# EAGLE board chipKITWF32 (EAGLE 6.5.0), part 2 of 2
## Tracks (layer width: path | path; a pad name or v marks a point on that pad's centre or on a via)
AN2/C2IN-/CN4/RB2
  Bottom 0.203: R24.2 65.53,7.37 70.36,2.54 70.61,2.54 J8.1
AN3/C2IN+/CN5/RB3
  Bottom 0.203: R25.2 66.67,7.49 69.22,4.95 70.99,4.95 J8.2
AN4/C1IN-/CN6/RB4
  Bottom 0.203: R26.2 67.82,7.49 69.09,6.22 69.22,6.22 71.5,6.22 72.39,5.33 72.39,3.81 J8.3
AN5/C1IN+/VBUSON/CN7/RB5
  Top 0.127: JP11.2 71.37,15.24 74.55,12.06 75.82,12.06 76.45,11.43 76.45,10.16 76.71,9.91 76.71,8.13 J8.4
  Bottom 0.127: R27.2
  Bottom 0.203: R27.2 68.96,7.24 69.6,6.6 71.75,6.6 73.28,5.08 J8.4
AN8/C1OUT/RB8
  Bottom 0.203: R28.2 70.1,7.49 70.61,6.99 72.01,6.99 72.77,6.22 74.17,6.22 74.93,5.46 74.93,3.81 J8.5
AN9/C2OUT/RB9
  Bottom 0.203: R29.2 71.75,7.37 72.26,7.37 73.03,6.6 74.68,6.6 J8.6
AN10/CVREFOUT/PMA13/RB10
  Bottom 0.203: R30.2 53.84,11.93 JP4.1
AN11/PMA12/RB11
  Bottom 0.203: R31.2 53.84,8.39 JP5.1
AN13/PMA10/RB13  (via drill 0.23 pad 0.43)
  Top 0.203: IC2.42 55.7,21.79 55.63,21.72 55.63,20.19 57.02,18.8 v61.34,18.8 | v67.06,20.83 70.36,20.83 71.12,21.59 71.12,25.65 71.5,26.04 71.5,32.38 v72.14,33.02
  Bottom 0.203: v61.34,18.8 64.39,18.8 66.42,20.83 v67.06,20.83 | v72.14,33.02 72.38,33.02 R35.1
AN14/PMALH/PMA1/RB14
  Bottom 0.203: R33.2 76.2,7.37 77.6,7.37 78.23,6.73 79.63,6.73 J8.10
AN15/OCFB/PMALL/PMA0/CN12/RB15
  Bottom 0.203: R34.2 79.75,7.88 81.41,6.22 82.68,6.22 J8.12
AVCC
  Top 0.254: IC2.30 50.9,21.94 C16.1
  pour Top (no thermals): 50.29,21.46 50.29,19.81 47.88,19.81 47.88,20.95 49.02,20.95 49.53,21.46
D+/RG2  (via drill 0.23 pad 0.43)
  Top 0.203: v83.06,17.65 82.93,17.53 76.69,17.53 J13.3 75.71,17.53 75.06,17.53 72.77,19.81 66.67,19.81 64.52,21.97 64.52,26.29 63.5,27.3 61.85,27.3 61.61,27.06 IC2.57
  Bottom 0.203: J12.3 83.69,17.02 v83.06,17.65
D-/RG3  (via drill 0.23 pad 0.43)
  Top 0.203: v83.82,17.65 83.19,17.02 77.2,17.02 J13.2 75.07,17.14 74.8,17.14 72.52,19.43 66.42,19.43 64.14,21.72 64.14,26.04 63.25,26.92 61.98,26.92 61.72,26.66 IC2.56
  Bottom 0.203: J12.2 83.83,17.67
  Bottom 0.254: 83.83,17.67 v83.82,17.65
FT3V3  (via drill 0.23 pad 0.43)
  Top 0.508: 12.32,25.02 12.32,22.61 12.95,21.97 14.86,21.97 v16.26,20.57 | 12.32,25.02 12.57,25.27 12.57,26.8 11.94,27.43 11.94,29.59 12.83,30.48 v15.75,30.48 v16.76,30.48 | 12.32,25.02 11.05,25.02 v10.16,25.91
  Bottom 0.127: R3.2 v16.76,30.48 | R5.2 v15.75,30.48
  Bottom 0.254: IC1.16 10.96,25.63 C6.1 v10.17,25.92 v10.16,25.91 | IC1.1 15.72,20.59 C5.1 16.25,20.57 v16.26,20.57
GND  (via drill 0.23 pad 0.43)
  Top 0.127: C20.2 63,34.55 v62.99,34.54 | C19.2 v63,37.58 v62.99,37.59
  Top 0.254: IC3.30 22.35,31.5 22.1,31.24 C23.2 21.84,30.23 v21.84,29.97 | IC3.18 8.38,51.94 8.64,51.69 v8.64,51.56 | IC3.10 v18.54,51.44 | IC3.1 v29.97,51.44 | IC3.19 v8.38,32.38 | IC3.25 v16,32.38 | IC3.28 v19.81,32.38 | IC3.36 v29.97,32.38 | C16.2 | C16.2 51.05,20.58 v51.05,20.57 | C15.2 51.05,19.93 v50.8,19.68 | C16.2 51.05,21.45 51.3,21.71 IC2.31 | IC2.36 53.3,21.63 53.47,21.46 53.47,21.09 C11.2 53.48,20.58 v53.47,20.57 | v57.28,20.7 57.28,20.83 C12.2 56.9,21.21 IC2.45 | IC2.15 46,28.66 C10.2 45.47,28.7 v45.21,28.7 | C9.2 v45.22,35.04 v45.21,35.05 | IC2.65 59.85,30.26 v59.82,30.23 | C13.2 62.49,27.95 62.74,28.19 v62.99,28.19 | C7.2 62.6,25.53 v62.99,25.53 | IC2.75 60.8,34.51 v60.83,34.54 | v19.94,3.68 19.47,4.15 J11.6
  Top 1.27: 5.08,20.19 J1.S3 J1.S2 5.08,29.09 | 5.08,20.19 J1.S4 | J1.S1 5.08,29.09 | J1.S5 5.08,29.09 | J1.S6 5.08,20.19
  Route2 1.524: 4.32,12.19 J17.2 4.32,4.45 5.84,2.92 J17.3
  Bottom 0.127: C2.2 R6.1 v10.67,29.46 | R47.1 v23.37,25.4 | R48.1 v32.77,25.4 | R45.1 v13.2,51.3 v13.21,51.31 | R58.1 v79.49,15.76 v79.5,15.75 | C18.2 62.37,28.71 v61.98,28.32 | C17.2 62.62,33.77 v62.99,33.4
  Bottom 0.203: Q2.1 v79.12,42.55 | Q2.4 80.45,44.13 v80.52,44.2
  Bottom 0.254: IC1.24 15.72,26.52 v15.88,26.67 | IC1.26 16.74,25.13 v16.76,25.15 | C6.2 v10.17,26.92 v10.16,26.92 | IC1.4 v14.22,21.09 v14.22,21.08 | C5.2 16,19.81 v16.13,19.81 | IC1.17 11.97,26.13 v11.81,26.29 | R65.1 v35.31,22.1 | IC1.20 13.72,26.94 C4.2 13.96,27.68 v13.97,27.69 | C3.2 14.35,28.7 | 14.35,28.7 v13.97,28.32 | C24.2 v8.64,51.55 v8.64,51.56 | D2.2 v31.5,41.02 | R62.1 31.11,8.89 v31.88,8.13 | 14.35,28.7 14.35,28.83 14.1,29.08 v13.97,29.08 | D1.1 49.67,30.37 v49.4,30.1 | Q1.1 v83.19,42.55 | Q1.4 84.52,44.13 v84.58,44.2 | C14.2 53.59,37.08 v53.59,37.34 | C8.2 57.64,36.97 v57.28,37.34 | v19.68,48.77 19.68,49.13 C21.2 18.92,49.16 v18.92,48.77 | v4.7,33.53 4.7,33.92 C22.2 5.08,34.29 5.46,33.91 v5.46,33.53 | C25.2 20.07,3.55 v19.94,3.68
  Bottom 1.27: J12.S3 J12.S1 J12.S2 J12.S4 87.25,13.27 v87.25,11.18
  other vias: 6.48,22.48 6.99,21.97 85.22,15.24 84.2,15.24 13.21,24.64 14.73,24.64 13.21,23.11 14.73,23.11 7.49,22.48 8,21.97 8.51,22.48 13.34,10.92 13.34,11.94 13.34,12.95 13.34,13.72 13.34,14.61 14.22,10.92 14.22,11.94 14.22,12.95 22.73,7.24 22.73,6.48 23.75,6.48 32.26,20.45 32.77,20.07 33.4,20.45 33.15,17.78 34.04,17.78 36.83,17.91 36.07,17.91 37.85,14.99 37.85,13.97 35.31,17.91 37.34,14.48 37.34,13.34 37.85,12.95 37.34,12.32 82.8,22.35 82.8,21.72 83.57,15.75 83.57,14.61 84.84,14.61 81.03,14.22 81.03,13.34 80.52,18.54 81.92,18.54 86.87,11.81 87.63,11.81
  pour Top (no thermals): 6.22,23.37 9.02,23.37 9.02,21.72 6.22,21.72
  pour Bottom (no thermals): 85.47,16 83.06,16 83.06,14.22 85.47,14.22
  pour Top (no thermals): 5.21,5.59 5.21,9.65 4.7,10.16 3.94,10.16 3.43,9.65 3.43,5.59 3.94,5.08 4.7,5.08
  pour Top (no thermals): 5.33,2.03 9.4,2.03 9.91,2.54 9.91,3.3 9.4,3.81 5.33,3.81 4.83,3.3 4.83,2.54
  pour Bottom (no thermals): 3.43,9.65 3.94,10.16 4.7,10.16 5.21,9.65 5.21,5.59 4.7,5.08 3.94,5.08 3.43,5.59
  pour Bottom (no thermals): 4.83,3.3 5.33,3.81 9.4,3.81 9.91,3.3 9.91,2.54 9.4,2.03 5.33,2.03 4.83,2.54
  pour Bottom (no thermals): 13.08,9.27 15.11,9.27 15.11,14.99 13.08,14.99
  pour Bottom (no thermals): 22.48,7.49 22.61,7.62 24,7.62 24,5.59 22.48,5.59
  pour Bottom (no thermals): 32,22.48 32,19.81 32.77,19.81 32.89,19.68 32.89,17.14 37.21,17.14 37.34,17.02 37.34,14.73 37.21,14.61 35.05,14.61 35.05,12.19 38.61,12.19 38.61,18.29 37.08,19.81 35.18,19.81 35.18,18.41 34.92,18.16 33.78,18.16 33.66,18.29 33.66,22.48
  pour Route2: 12.57,0 12.57,11.18 0,11.18 0,35.94 11.81,35.94 11.81,50.93 8.26,50.93 8.26,53.34 88.9,53.34 88.9,0
  pour Route2 (no thermals): 3.43,9.65 3.94,10.16 4.7,10.16 5.21,9.65 5.21,5.59 4.7,5.08 3.94,5.08 3.43,5.59
  pour Route2 (no thermals): 4.83,2.54 4.83,3.3 5.33,3.81 9.4,3.81 9.91,3.3 9.91,2.54 9.4,2.03 5.33,2.03
  pour Bottom (no thermals): 82.55,22.61 82.55,21.59 83.82,21.59 83.82,22.61
  pour Bottom (no thermals): 80.64,14.73 80.64,12.7 82.55,12.7 82.55,14.73
  pour Bottom (no thermals): 80.14,18.92 80.14,18.16 82.17,18.16 82.17,18.92
  pour Route15 (no thermals): 5.21,5.59 5.21,9.65 4.7,10.16 3.94,10.16 3.43,9.65 3.43,5.59 3.94,5.08 4.7,5.08
  pour Route15 (no thermals): 5.33,2.03 9.4,2.03 9.91,2.54 9.91,3.3 9.4,3.81 5.33,3.81 4.83,3.3 4.83,2.54
IC4/PMCS1/PMA14/RD11  (via drill 0.23 pad 0.43)
  Top 0.127: IC2.71 59.66,32.66 v59.31,33.02 59.05,33.27 59.05,34.04 60.07,35.05 60.2,35.05 61.34,36.2 61.34,36.45 61.59,36.7 61.59,37.85 62.99,39.24 v62.99,42.93
  Bottom 0.127: v59.31,33.02 59.17,33.02 R13.2 | J7.4 59.44,48.64 60.33,49.53 62.23,49.53 62.99,48.77 v62.99,42.93
IC5/PMD12/RD12
  Top 0.127: IC2.79 57.7,37.13 57.78,37.21 57.78,37.85 R15.1
INT1/RE8  (via drill 0.23 pad 0.43)
  Top 0.127: IC2.18 50.45,27.46 v51.69,28.7
  Bottom 0.127: v51.69,28.7 51.82,28.57 52.45,28.57 52.7,28.83 53.21,28.83 53.59,29.21 55.37,29.21 56.9,30.73 R16.2 58.42,30.23 59.18,30.23 59.44,30.48 59.44,30.61 59.69,30.86 60.2,30.86 60.83,30.23 60.83,28.19 62.36,26.67 63.5,26.67 64.26,25.91 67.82,25.91 68.71,26.8 68.71,30.61 70.1,32 72.52,32 73.41,32.89 73.41,34.42 73.66,34.67 73.66,36.2 74.93,37.47 74.93,44.83 77.6,47.5 77.6,49.66 J9.5
INT2/RE9  (via drill 0.23 pad 0.43)
  Top 0.127: IC2.19 51.07,27.06 52.2,28.19 v52.2,29.08 | v59.69,33.53 59.69,34.29 60.07,34.67 60.33,34.67 61.98,36.32 61.98,37.34 63.75,39.12 63.75,42.67 v64.39,43.31
  Bottom 0.127: v52.2,29.08 52.32,29.21 53.09,29.21 53.47,29.59 55.24,29.59 57.4,31.75 R17.2 58.42,32.26 58.42,33.15 58.8,33.53 v59.69,33.53 | v64.39,43.31 64.39,49.15 J9.15
MISO
  Top 0.127: J10.1 80.77,30.48 79.63,31.62 76.2,31.62 74.8,30.23 74.8,28.32 JP6.2
MOSI
  Top 0.127: J10.4 86.36,28.57 85.72,29.21 81.15,29.21 79.76,30.61 79.63,30.61 79.25,30.99 77.22,30.99 JP7.2
N$1  (via drill 0.23 pad 0.43)
  Top 0.203: IC2.25 46.51,24.66 46.23,24.38 46.23,20.19 50.04,16.38 60.33,16.38 64.39,12.32 69.09,12.32 69.72,11.68 69.72,11.43 70.1,11.05 v71.37,11.05
  Bottom 0.203: R22.1 72.27,8.88 71.75,9.4 71.63,9.4 71.37,9.65 v71.37,11.05 71.63,11.3 D5.4
N$2  (via drill 0.23 pad 0.43)
  Top 0.203: IC2.24 46.27,25.06 45.72,24.51 45.72,19.81 49.66,15.88 59.94,15.88 64.01,11.81 68.96,11.81 69.22,11.56 69.22,10.92 70.23,9.91 71.44,9.91 D5.5 v72.77,10.67
  Bottom 0.203: D5.5 v72.77,10.67 72.9,10.54 72.9,9.52 R23.1
N$3  (via drill 0.23 pad 0.43)
  Top 0.203: IC2.23 45.91,25.46 45.21,24.77 45.21,19.43 49.28,15.37 59.56,15.37 63.75,11.18 v64.9,11.18
  Bottom 0.203: 66.04,10.03 65.53,9.53 R24.1 | v64.9,11.18 65.02,11.05 65.02,10.41 65.28,10.16 65.91,10.16 66.04,10.03 | D4.1 66.04,10.03
N$4  (via drill 0.23 pad 0.43)
  Top 0.203: IC2.22 45.68,25.86 44.7,24.89 44.7,19.18 49.02,14.86 59.18,14.86 63.37,10.67 v65.53,10.67
  Bottom 0.203: R25.1 66.93,9.14 66.93,10.41 66.67,10.67 D4.2 v65.53,10.67
N$5  (via drill 0.23 pad 0.43)
  Top 0.203: IC2.21 45.31,26.26 44.2,25.15 44.2,18.8 48.64,14.35 58.67,14.35 62.99,10.03 66.93,10.03 68.2,11.3 v68.71,11.3
  Bottom 0.203: R26.1 67.44,9.27 67.44,11.05 67.56,11.18 68.01,11.18 D4.4 v68.71,11.3
N$6  (via drill 0.23 pad 0.43)
  Top 0.203: IC2.20 44.95,26.66 43.69,25.4 43.69,18.29 48.26,13.72 58.29,13.72 62.48,9.53 67.06,9.53 68.2,10.67 v68.71,10.67
  Bottom 0.203: R27.1 68.96,10.41 v68.71,10.67 D4.5
N$7  (via drill 0.23 pad 0.43)
  Top 0.127: IC2.64 60.82,29.84 61.59,29.84 v62.1,30.35
  Bottom 0.127: R36.2 v62.1,30.35
N$8
  Bottom 0.127: X1.1 67.39,33.73 65.28,31.62 64.01,31.62 62.87,32.77 62.49,32.77 C17.1 R36.1
N$9  (via drill 0.23 pad 0.43)
  Top 0.203: 51.69,22.78 IC2.32 51.7,21.48 51.56,21.34 51.56,19.56 54.23,16.89 60.96,16.89 65.02,12.83 v65.41,12.83
  Bottom 0.203: v65.41,12.83 67.94,12.83 69.22,11.56 69.22,10.79 69.47,10.54 69.47,10.29 69.72,10.03 D5.1 70.29,9.07 R28.1
N$10  (via drill 0.23 pad 0.43)
  Top 0.203: IC2.33 52.1,21.37 52.07,21.34 52.07,19.81 54.48,17.4 61.59,17.4 65.66,13.34 v65.91,13.34
  Bottom 0.203: R29.1 70.99,9.14 70.99,10.41 70.74,10.67 D5.2 69.85,10.67 69.6,10.92 69.6,11.81 68.07,13.34 v65.91,13.34
N$11  (via drill 0.23 pad 0.43)
  Top 0.203: 52.5,25.07 v52.7,25.27 52.2,24.77 52.2,24.51 52.5,24.21 IC2.34 52.5,20.14 54.74,17.91 v55.12,17.91
  Bottom 0.127: R30.1 52.84,13.22 52.83,13.21
  Bottom 0.203: v52.7,25.27 53.28,25.27 D3.4 | v55.12,17.91 55.12,15.61 R30.1
N$12  (via drill 0.23 pad 0.43)
  Top 0.203: v52.83,24.64 52.9,24.57 IC2.35 52.9,20.5 54.86,18.54 55.5,18.54 55.88,18.16 v55.88,17.91
  Bottom 0.203: D3.5 52.96,24.77 v52.83,24.64 | R31.1 52.07,8.14 52.07,9.78 52.45,10.16 54.23,10.16 54.61,10.54 54.61,12.57 55.88,13.84 v55.88,17.91
N$13  (via drill 0.23 pad 0.43)
  Top 0.203: v32.89,11.05 33.27,11.43 50.67,11.43 52.2,12.95 56.52,12.95 57.15,12.32 57.15,11.05 57.91,10.29 60.07,10.29 61.59,8.76 74.55,8.76 75.95,10.16 75.95,10.92 v75.56,11.3 | v69.72,12.45 68.83,13.34 66.8,13.34 61.98,18.16 56.9,18.16 55.12,19.94 55.12,21.72 55.3,21.9 IC2.41
  Bottom 0.203: R32.1 v32.89,11.05 | D6.4 v75.56,11.3 74.55,12.32 69.85,12.32 v69.72,12.45
N$14  (via drill 0.23 pad 0.43)
  Top 0.127: v29.34,36.58 26.29,36.58 v23.62,33.91
  Bottom 0.127: C1.2 17.78,23.87 17.78,29.46 22.23,33.91 v23.62,33.91 | JP1.2 39.37,34.29 36.96,34.29 35.69,35.56 30.35,35.56 v29.34,36.58
N$15  (via drill 0.23 pad 0.43)
  Top 0.203: IC2.43 56.1,21.68 56.01,21.59 56.01,20.45 57.15,19.3 61.98,19.3 67.44,13.84 69.09,13.84 70.99,11.94 72.39,11.94 v73.66,10.67
  Bottom 0.203: R33.1 75.18,9.39 75.18,10.03 74.93,10.29 74.93,10.41 74.68,10.67 D6.2 v73.66,10.67
N$16  (via drill 0.23 pad 0.43)
  Top 0.203: IC2.44 56.5,21.58 56.39,21.46 56.39,20.7 57.28,19.81 62.61,19.81 68.07,14.35 69.34,14.35 71.25,12.45 73.41,12.45 74.42,11.43 74.55,11.43 v75.31,10.67
  Bottom 0.203: R34.1 76.83,10.41 76.58,10.67 D6.5 v75.31,10.67
N$17  (via drill 0.23 pad 0.43)
  Top 0.127: IC2.63 61.85,29.46 v61.98,29.59
  Bottom 0.127: X1.3 64.69,28.24 65.66,29.21 65.66,30.86 65.28,31.24 64.01,31.24 63.5,30.73 63.5,29.97 63.25,29.72 62.49,29.72 | 62.49,29.72 C18.1 | 62.49,29.72 62.1,29.72 v61.98,29.59
N$18
  Top 0.127: X2.2 65.79,36.7 65.41,37.08 64.9,37.08 64.64,36.83 64.64,36.2 64.26,35.81 63.76,35.81 C20.1 62.99,35.05 62.87,35.05 62.36,34.54 62.36,33.91 61.91,33.46 IC2.73
N$19
  Top 0.127: IC2.74 61.8,33.86 61.98,34.04 61.98,34.8 62.23,35.05 62.23,35.31 R37.2
N$20
  Top 0.127: X2.1 65.79,37.85 65.41,37.47 64.77,37.47 64.26,36.96 64.26,36.32 64.14,36.2 63.88,36.2 C19.1 62.5,36.58 R37.1
N$21  (via drill 0.23 pad 0.43)
  Top 0.127: IC2.13 v46.23,29.46
  Bottom 0.127: D1.3 46.48,29.72 v46.23,29.46 45.97,29.46 R8.1
N$22
  Bottom 0.127: R56.2 79.63,44.58 79.63,43.43 79.88,43.18 Q2.5
N$23
  Bottom 0.127: Q2.3 77.85,43.81 77.6,43.56 77.6,40.64 78.49,39.75 79.5,39.75 79.76,40.01 79.76,40.64 R51.1
N$24  (via drill 0.23 pad 0.43)
  Top 0.254: IC2.85 55.3,37.41 v55.24,37.47
  Bottom 0.254: C8.1 55.24,36.97 v55.24,37.47
N$25
  Bottom 0.127: R54.1 82.04,16.26 82.04,16.89 81.34,17.59 IC4.3 80.33,17.59 79.63,18.29 77.6,18.29 76.58,19.3 69.98,19.3 JP9.1
N$26  (via drill 0.23 pad 0.43)
  Top 0.127: v80.9,40.77 80.9,41.01 LD5.C
  Bottom 0.127: R51.2 v80.9,40.77
N$27
  Bottom 0.127: R9.1 39.38,38.61 38.2,38.61 BTN1.1B BTN1.2B
N$28  (via drill 0.23 pad 0.43)
  Top 0.127: LD6.C 78.75,41.39 79.12,41.02 v79.12,40.77
  Bottom 0.127: v79.12,40.77 v79.11,40.77 R52.2
N$29  (via drill 0.23 pad 0.43)
  Top 0.127: IC3.26 17.27,31.75 16.89,32.13 v16.89,32.51
  Bottom 0.127: v16.89,32.51 16.89,32.65 R38.1
N$30
  Bottom 0.127: J16.5 49.28,7.37 R63.2
N$31
  Bottom 0.127: Q2.2 79.12,43.18 79.25,43.31 79.25,44.7 R57.2
N$32
  Bottom 0.127: 80.26,42.55 Q2.6 80.39,42.55 79.24,41.39 R52.1
N$33  (via drill 0.23 pad 0.43)
  Top 0.254: J1.2 9.11,25.44 v9.14,25.4
  Bottom 0.254: IC1.15 9.93,25.13 9.65,25.4 v9.14,25.4
N$34
  pour Bottom (no thermals): 23.62,17.65 23.62,14.61 28.7,14.61 30.99,12.32 33.02,12.32 33.02,14.61 32.64,14.61 32.64,16.64 31.5,16.64 31.24,16.38 30.23,16.38 29.97,16.64 29.97,17.4 29.72,17.65
N$35
  Bottom 0.305: 30.75,16.89 C30.1 D8.C | 32.32,18.73 31.88,18.29 30.75,18.29
  Bottom 0.508: IC6.1 32.32,18.73 | 30.75,18.29 D8.C
N$36
  pour Bottom (no thermals): 20.57,6.86 22.1,6.86 22.1,7.62 22.48,8 24,8 24,10.29 22.86,10.29 22.86,9.53 22.61,9.27 20.57,9.27
N$37  (via drill 0.23 pad 0.43)
  Top 0.254: J1.3 9.14,24.64 v9.27,24.77
  Bottom 0.254: IC1.14 9.41,24.63 v9.27,24.77
N$38
  Bottom 0.254: IC6.3 34.22,19.62 34.29,19.68 R64.1 R65.2
N$39
  pour Bottom (no thermals): 17.78,3.56 17.78,8.64 17.4,9.02 13.08,9.02 13.08,3.56
N$40
  Bottom 0.203: R35.2 VR1.2
N$41
  Bottom 0.127: IC1.30 18.02,23.13 18.29,22.86 18.29,22.34 R1.1
N$43
  Bottom 0.127: IC1.2 15.22,21.06 15.11,20.95 15.11,19.18 15.49,18.8 R2.1
N$45  (via drill 0.23 pad 0.43)
  Top 0.127: IC3.16 10.92,52.07 v11.81,51.18
  Bottom 0.127: v11.81,51.18 v11.82,51.18 R45.2
N$46
  Top 0.203: J8.9 80.01,1.27 70.1,1.27 64.52,6.86 58.67,6.86 57.15,8.38 57.15,10.16 JP4.2
N$47
  Bottom 0.127: IC1.18 12.72,26.4 12.19,26.92 12.19,27.44 C2.1 R6.2 9.67,28.95 R4.1
N$48  (via drill 0.23 pad 0.43)
  Top 0.127: IC2.28 50.1,24.19 50.67,24.77 v50.93,24.77 51.05,24.77 51.44,25.15 51.44,26.67 52.7,27.94 52.7,29.34 52.45,29.59 v50.93,29.59
  Bottom 0.127: v50.93,24.77 D3.2 | R20.1 45.47,38.35 43.43,36.32 42.8,36.32 42.42,35.94 42.42,35.18 42.55,35.05 42.55,30.86 44.2,29.21 45.59,29.21 45.85,28.96 46.74,28.96 46.99,29.21 48.77,29.21 49.15,29.59 v50.93,29.59
N$49
  Top 0.203: J8.11 82.04,0.76 69.85,0.76 64.52,6.1 58.67,6.1 JP5.2
N$50
  Bottom 0.127: JP3.2 56.13,41.53 55.37,42.29 55.37,47.24 55.75,47.62 55.75,49.66 J7.5
N$51  (via drill 0.23 pad 0.43)
  Top 0.127: LD4.C 82.68,41.02 v82.68,40.77
  Bottom 0.127: v82.68,40.77 82.67,40.77 R50.2
N$52
  Bottom 0.127: IC1.8 12.22,20.73 10.54,19.05 7.87,19.05 J2.1
N$53
  Bottom 0.127: IC1.31 17.51,22.63 C1.1
N$54
  Bottom 0.127: IC1.6 13.22,18.43 12.7,17.91 12.7,16.76 12.06,16.13 9.78,16.13 J2.2
N$55
  Bottom 0.127: IC1.7 12.72,18.56 11.43,17.27 J2.3
N$56
  Bottom 0.127: IC1.3 14.72,17.77 14.22,17.27 J2.4
N$57  (via drill 0.23 pad 0.43)
  Top 0.127: v15.75,27.56 15.86,27.56 LD1.C
  Bottom 0.127: IC1.22 14.72,26.53 v15.75,27.56
N$58  (via drill 0.23 pad 0.43)
  Top 0.127: v14.99,27.56 LD2.C
  Bottom 0.127: IC1.21 14.22,26.54 14.99,27.3 v14.99,27.56
N$59  (via drill 0.23 pad 0.43)
  Top 0.127: v17.14,29.34 16.88,29.34 LD1.A
  Bottom 0.127: R3.1 16.77,28.96 v17.14,29.34
N$60  (via drill 0.23 pad 0.43)
  Top 0.127: v15.37,29.21 15.37,29.32 LD2.A
  Bottom 0.127: R5.1 15.61,28.96 v15.37,29.21
N$61  (via drill 0.23 pad 0.43)
  Top 0.127: IC2.29 50.5,23.83 50.8,24.13 v50.93,24.13 51.18,24.13 51.56,24.51 51.56,24.77 52.07,25.27 52.07,26.29 53.09,27.3 53.09,29.59 v52.96,29.72
  Bottom 0.127: v50.93,24.13 D3.1 | v52.96,29.72 51.69,29.72 51.18,29.21 51.18,28.96 50.8,28.57 47.24,28.57 46.1,27.43 44.83,27.43 42.04,30.23 42.04,36.07 42.67,36.7 43.31,36.7 44.83,38.23 44.83,43.69 44.45,44.07 R21.1
N$62
  Bottom 0.127: IC4.4 78.49,17.28 R58.2 77.85,16.26 77.6,16 77.6,15.49 76.96,14.86 74.68,14.86 JP11.1
N$63  (via drill 0.23 pad 0.43)
  Top 0.127: LD3.C 84.09,41.39 84.45,41.02 v84.45,40.77
  Bottom 0.127: v84.45,40.77 R49.2
N$64
  Bottom 0.127: Q1.6 84.33,42.55 83.82,42.04 82.94,42.04 R50.1
N$65
  Bottom 0.127: Q1.3 82.17,43.81 81.92,43.56 81.92,42.42 81.53,42.04 81.53,40.13 81.92,39.75 82.93,39.75 83.19,40.01 83.19,40.51 R49.1
N$66
  Bottom 1.016: J13.1 78.47,13.52 C27.1
  pour Route15 (no thermals): 71.75,23.11 71.12,22.48 71.12,20.95 73.03,19.05 73.03,14.73 75.18,12.57 76.96,12.57 76.96,14.48 75.95,14.48 75.31,15.11 75.31,19.68 73.79,21.21 73.79,22.48 73.15,23.11
N$67
  Bottom 0.127: Q1.2 83.06,43.18 83.31,43.43 83.31,44.7 R55.2
N$68
  pour Bottom (no thermals): 68.45,22.73 68.45,21.34 68.71,21.08 70.74,21.08 71.12,21.46 71.12,22.61 71.75,23.24 74.8,23.24 77.6,20.45 80.01,20.45 80.64,19.81 80.64,19.18 81.66,19.18 81.66,20.95 82.17,21.46 82.17,22.48 81.41,22.48 81.41,21.72 81.15,21.46 77.72,21.46 75.18,24 69.72,24
N$69
  Bottom 0.127: R53.2 83.69,44.58 83.69,43.43 83.95,43.18 Q1.5
N$71
  Bottom 0.127: 32.74,23.91 R48.2 | R48.2 R44.2 33.81,23.91 BTN2.2A | BTN2.1A 29.29,23.88 R48.2
N$72  (via drill 0.23 pad 0.43)
  Top 0.127: v22.73,23.88 19.9,23.88 BTN3.1A
  Bottom 0.127: v22.73,23.88 22.77,23.91 23.34,23.91 R47.2 R46.2 24.41,23.91 BTN3.2A
OC2/RD1  (via drill 0.23 pad 0.43)
  Top 0.127: IC2.76 58.9,36.93 59.18,37.21 v59.18,39.12
  Bottom 0.127: J9.11 69.85,49.53 69.85,47.62 69.22,46.99 69.22,43.94 66.55,41.27 63.12,41.27 61.09,39.24 59.31,39.24 v59.18,39.12
OC3/RD2  (via drill 0.23 pad 0.43)
  Top 0.127: IC2.77 58.5,37.04 58.8,37.34 58.8,38.73 58.67,38.86 58.67,39.75 v59.18,40.26
  Bottom 0.127: v59.18,40.26 59.31,40.26 59.56,40.01 60.33,40.01 62.36,42.04 65.41,42.04 66.55,43.18 66.55,46.74 67.31,47.5 67.31,49.53 J9.13
OC4/RD3  (via drill 0.23 pad 0.43)
  Top 0.127: IC2.78 58.1,37.02 58.42,37.34 58.42,38.48 57.66,39.24 57.66,42.55 v57.4,42.8
  Bottom 0.127: J7.3 59.31,50.8 58.17,49.66 58.17,43.56 v57.4,42.8
OC5/PMWR/CN13/RD4
  Top 0.127: JP3.1 54.86,42.67 56.77,42.67 57.28,42.16 57.28,38.99 56.9,38.62 R15.2 56.77,37.84 56.77,37.21 56.9,37.08 IC2.81
P32_PGC  (via drill 0.23 pad 0.43)
  Top 0.127: IC2.26 49.3,21.87 v49.28,21.84 | v37.85,25.27 37.85,30.48 35.56,32.77 35.56,35.1 JP2.5
  Bottom 0.127: D2.5 30.85,39.64 33.27,37.21 33.45,37.21 JP2.5 | v49.28,21.84 41.02,21.84 37.85,25.02 v37.85,25.27
P32_PGD  (via drill 0.23 pad 0.43)
  Top 0.127: JP2.4 34.42,39.37 36.2,37.59 36.2,33.02 38.35,30.86 v38.35,25.65 | v48.64,23.5 49.02,23.88 49.4,23.88 49.7,23.58 IC2.27
  Bottom 0.127: D2.4 33.87,39.74 JP2.4 | v38.35,25.65 38.35,25.4 40.39,23.37 47.24,23.37 47.37,23.5 v48.64,23.5
P32_RST  (via drill 0.23 pad 0.43)
  Top 0.127: v37.34,23.75 39.5,25.91 39.5,32.38 38.1,33.78 JP1.1 38.1,36.32 38.61,36.83 41.78,36.83 v42.93,35.69
  Bottom 0.127: JP2.1 32.38,45.54 32.38,41.91 32.15,41.67 D2.3 32.15,41.51 33.02,40.64 35.94,40.64 36.45,40.13 36.45,37.21 JP1.1 38.61,35.56 38.73,35.69 38.73,36.97 R9.2 R7.1 | v37.34,23.75 37.34,21.21 40.64,17.91 40.64,17.78 46.61,11.81 46.61,9.27 46.86,9.02 46.86,6.6 48.9,4.57 50.8,4.57 52.83,2.54 J3.3 | R8.2 44.32,30.1 44.07,30.1 43.05,31.11 43.05,35.56 v42.93,35.69
PGEC1/AN1/CN3/RB1
  Bottom 0.203: R23.2 73.91,7.49 75.06,7.49 75.69,6.86 76.96,6.86 J8.8
PGED1/AN0/CN2/RB0
  Bottom 0.203: R22.2 73.28,6.99 74.93,6.99 75.56,6.35 76.58,6.35 77.34,5.59 77.34,3.94 J8.7
PMD0/RE0
  Top 0.127: J9.2 81.79,46.23 78.11,46.23 76.45,44.58 54.74,44.58 50.93,40.77 50.93,38.23 52.1,37.05 IC2.93
PMD1/RE1
  Top 0.127: J9.4 79.63,46.61 77.85,46.61 76.33,45.09 54.61,45.09 50.55,41.02 50.55,38.1 51.7,36.94 IC2.94
PMD2/RE2
  Top 0.127: IC2.98 50.1,41.21 54.48,45.59 76.07,45.59 77.22,46.74 77.47,46.74 78.74,48.01 J9.6
PMD3/RE3
  Top 0.127: IC2.99 49.7,41.07 49.7,41.45 49.78,41.53 54.36,46.1 54.74,46.1 74.8,46.1 76.2,47.5 J9.8
PMD4/RE4
  Top 0.127: IC2.100 49.3,41.68 49.4,41.78 54.23,46.61 73.03,46.61 73.66,47.24 J9.10
PMD5/RE5  (via drill 0.23 pad 0.43)
  Top 0.127: IC2.3 48.2,33.46 48.77,34.04 51.18,34.04 v51.82,34.67
  Bottom 0.127: v51.82,34.67 52.07,34.42 52.83,34.42 53.21,34.8 53.21,35.05 53.85,35.69 58.55,35.69 62.1,39.24 62.23,39.24 63.5,40.51 67.44,40.51 70.74,43.81 70.74,47.88 J9.12
PMD6/RE6  (via drill 0.23 pad 0.43)
  Top 0.127: IC2.4 48.3,33.06 49.02,33.78 52.2,33.78 52.7,34.29 v52.7,34.92
  Bottom 0.127: v52.7,34.92 52.83,35.05 52.83,37.97 54.1,39.24 57.28,39.24 57.66,39.62 60.83,39.62 62.87,41.66 66.17,41.66 67.82,43.31 67.82,47.5 J9.14
PMD7/RE7  (via drill 0.23 pad 0.43)
  Top 0.127: IC2.5 48.41,32.66 49.15,33.4 54.36,33.4 54.86,33.91 56.9,33.91 57.15,34.16 58.04,34.16 59.69,35.81 59.69,40.13 v60.07,40.51
  Bottom 0.127: v60.07,40.51 61.98,42.42 64.26,42.42 65.15,43.31 65.15,47.37 J9.16
PMD8/RG0  (via drill 0.23 pad 0.43)
  Top 0.127: IC3.7 22.35,51.56 v22.1,51.31 22.1,51.05 22.61,50.55 27.18,50.55 29.46,48.26 34.8,48.26 35.94,47.12 39.24,47.12 40.89,45.47 40.89,43.94 41.27,43.56 48.26,43.56 v49.28,42.55 | IC2.90 53.3,36.99 53.09,37.21 53.09,38.86 51.82,40.13 v51.69,40.13
  Bottom 0.127: v22.1,51.31 R43.1 | v49.28,42.55 v51.69,40.13
PMD9/RG1  (via drill 0.23 pad 0.43)
  Top 0.127: IC3.20 v9.65,32.38 9.65,32.51 10.67,33.53 19.3,33.53 31.37,45.59 35.31,45.59 38.23,42.67 43.69,42.67 48.77,37.59 v48.77,36.32 | IC2.89 53.7,35.41 53.59,35.31 v53.59,34.54
  Bottom 0.127: v48.77,36.32 51.05,34.04 53.34,34.04 53.59,34.29 v53.59,34.54 | R40.1 v9.65,32.38
PMD10/RF1  (via drill 0.23 pad 0.43)
  Top 0.127: IC2.88 v54.1,35.18
  Bottom 0.127: J9.9 72.39,49.53 72.39,44.7 67.82,40.13 63.63,40.13 62.36,38.86 62.23,38.86 58.67,35.31 54.23,35.31 v54.1,35.18
PMD11/RF0  (via drill 0.23 pad 0.43)
  Top 0.127: IC2.87 54.5,36.94 54.1,37.34 v54.1,38.23 | v69.85,43.81 70.1,44.07 76.83,44.07 77.98,45.21 81.15,45.21 81.28,45.34 v81.41,45.34
  Bottom 0.127: v54.1,38.23 54.36,38.48 60.83,38.48 63.25,40.89 66.93,40.89 v69.85,43.81 | v81.41,45.34 v81.4,45.34 R56.1
PMD13/CN19/RD13  (via drill 0.23 pad 0.43)
  Top 0.127: IC2.80 57.3,35.03 v57.53,34.8 | v46.23,33.27 43.31,30.35 43.31,25.91 43.05,25.65 43.05,17.78 v44.07,16.76
  Bottom 0.127: v57.53,34.8 57.15,34.8 57.02,34.92 54.48,34.92 54.1,34.54 54.1,34.04 53.72,33.66 46.61,33.66 v46.23,33.27 | v44.07,16.76 44.07,16.38 50.29,10.16 50.29,9.91 50.29,9.65 50.29,7.37 R63.1
PMD14/CN15/RD6  (via drill 0.23 pad 0.43)
  Top 0.127: v56.01,40.13 56.01,37.21 56.1,37.12 IC2.83 56.1,35.27 55.88,35.05 55.24,35.05 v54.61,34.42
  Bottom 0.127: J7.6 56.9,42.16 57.28,41.78 57.28,41.02 56.39,40.13 v56.01,40.13 | R14.2 54.62,34.41 v54.61,34.42
PMD15/CN16/RD7  (via drill 0.23 pad 0.43)
  Top 0.127: IC2.84 55.7,37.03 55.75,37.08 55.75,37.59 54.36,38.99 53.59,38.99 51.82,40.77 v51.82,41.02
  Bottom 0.127: J7.8 54.36,47.88 51.56,45.09 51.56,41.27 v51.82,41.02
PMRD/CN14/RD5  (via drill 0.23 pad 0.43)
  Top 0.127: v56.64,34.42 56.5,34.56 IC2.82 56.5,37.1 56.39,37.21 56.39,38.99 56.77,39.37 v56.77,39.75
  Bottom 0.127: J7.2 61.85,48.26 59.69,46.1 59.69,44.07 57.66,42.04 57.66,40.26 57.15,39.75 v56.77,39.75 | R12.2 56.63,34.41 v56.64,34.42
RG15
  Top 0.127: IC2.1 46.63,34.26 46.35,34.54 44.83,34.54 42.29,32 42.29,22.48 36.83,17.02 30.1,17.02 28.37,15.29 28.37,5.13 25.65,2.41 19.3,2.41 18.29,3.43 18.29,4.89 J11.7
RTCC/IC1/RD8  (via drill 0.23 pad 0.43)
  Top 0.127: IC2.68 59.72,31.46 v59.69,31.5
  Bottom 0.127: v59.69,31.5 v59.68,31.5 R16.1
SCK1/IC3/PMCS2/PMA15/RD10  (via drill 0.23 pad 0.43)
  Top 0.127: IC2.70 59.68,32.26 59.44,32.51 59.05,32.51 58.67,32.13 58.67,30.86 58.04,30.23 57.66,30.23 v57.53,30.1
  Bottom 0.127: R11.1 v57.53,30.1
SCK2/U6TX/U3RTS/PMA5/CN8/RG6  (via drill 0.23 pad 0.43)
  Top 0.127: IC2.10 45.54,30.66 v44.96,31.24
  Bottom 0.127: v44.96,31.24 44.45,31.75 44.45,33.27 44.32,33.4 44.32,35.31 44.45,35.43 44.45,35.81 47.24,38.61 47.24,44.45 50.42,47.62 50.42,49.66 J7.11 49.28,51.31 50.55,52.58 84.45,52.58 85.85,51.18 85.85,48.13 84.33,46.61 82.93,46.61 82.17,45.85 78.87,45.85 R57.1 | 77.98,44.97 R57.1 | R57.1 77.09,44.06 77.09,39.5 78.87,37.72 78.87,33.66 81.66,30.86 81.66,30.1 J10.3
SCK3/U4TX/U1RTS/CN21/RD15  (via drill 0.23 pad 0.43)
  Top 0.127: IC2.48 58.1,23.69 57.78,24 57.28,24 56.77,24.51 56.77,26.04 55.63,27.18 55.63,30.1 54.86,30.86 54.48,30.86 54.1,30.48 54.1,30.35 v53.98,30.23
  Bottom 0.127: v53.98,30.23 51.31,30.23 50.67,30.86 48.51,30.86 48.01,30.35 44.58,30.35 43.43,31.5 43.43,35.81 46.1,38.48 46.1,47.62 J7.14
SCK4/U5TX/U2RTS/RF13  (via drill 0.23 pad 0.43)
  Top 0.127: IC3.34 27.43,30.86 v28.19,30.1 | IC2.39 54.5,26.78 v54.1,27.18
  Bottom 0.127: v28.19,30.1 30.61,30.1 31.24,29.46 37.97,29.46 41.91,25.53 48.26,25.53 49.4,26.67 53.47,26.67 53.98,27.18 v54.1,27.18
SCL1/INT3/RA14  (via drill 0.23 pad 0.43)
  Top 0.127: IC2.66 59.49,30.66 59.31,30.48 59.31,29.84 v59.44,29.72 59.18,29.46 58.04,29.46 57.78,29.21 57.78,28.32 57.02,27.56 56.39,27.56 56.13,27.81 56.13,30.99 58.17,33.02 58.17,33.53 60.83,36.2 60.83,36.58 61.21,36.96 61.21,41.91 62.74,43.43 63.5,43.43 v63.63,43.31 | v63.5,20.07 67.69,15.88 68.58,15.88 JP9.2
  Bottom 0.127: R11.2 v59.44,29.72 59.94,29.21 59.94,26.04 60.83,25.15 60.83,22.73 v63.5,20.07 | v63.63,43.31 63.75,43.43 63.75,49.02 J7.1
SCL2/RA2  (via drill 0.23 pad 0.43)
  Top 0.127: IC2.58 59.85,27.46 59.69,27.3 58.42,27.3 v58.29,27.18
  Bottom 0.127: R18.2 v58.29,27.18 58.55,26.92 58.55,26.16 59.69,25.02 59.69,14.73 57.15,12.19 57.15,10.16 JP5.3 | R18.2 57.52,27.57 57.15,27.94 57.15,28.19 56.77,28.57 56.26,28.57 56.13,28.45 53.59,28.45 52.96,27.81 48.26,27.81 47.12,26.67 43.05,26.67 38.1,31.62 34.04,31.62 32.38,33.27 29.34,33.27 26.42,36.2 26.42,43.05 32,48.64 34.67,48.64 34.8,48.51 36.83,48.51 J6.2
  Bottom 0.203: R18.2
SCL3/SDO3/U1TX/RF8  (via drill 0.23 pad 0.43)
  Top 0.127: v57.91,25.4 57.98,25.46 IC2.53 61.53,25.46 62.1,24.89 62.1,24.64 62.61,24.13 v63.37,24.13
  Bottom 0.127: R2.2 20.45,18.29 21.46,19.3 21.46,21.46 21.72,21.72 21.72,25.15 22.73,26.16 38.48,26.16 40.64,24 49.78,24 51.18,22.61 56.9,22.61 58.29,24 58.29,25.02 v57.91,25.4 | v63.37,24.13 66.93,24.13 68.96,26.16 68.96,27.94 69.47,28.45 71.25,28.45 71.63,28.83 71.63,30.61 73.28,32.26 73.79,32.26 76.83,35.31 76.83,37.85 75.69,38.99 75.69,44.83 77.72,46.86 79.25,46.86 80.01,47.62 80.01,49.53 J9.3
SCL4/SDO2/U3TX/PMA3/CN10/RG8  (via drill 0.23 pad 0.43)
  Top 0.127: IC2.12 48.41,29.86 49.91,31.37 51.56,31.37 52.07,31.88 v52.07,32.38 | v73.79,37.85 75.06,37.85 76.45,36.45 76.45,33.66 73.53,30.73 73.53,29.84 JP7.1
  Bottom 0.127: J7.7 53.34,49.78 53.34,47.5 48.77,42.93 48.77,38.35 46.1,35.69 46.1,33.91 45.59,33.4 45.59,33.15 45.97,32.77 48.77,32.77 49.28,32.26 50.16,32.26 50.29,32.38 v52.07,32.38 54.61,32.38 54.99,32 56.13,32 57.02,32.89 57.02,33.27 58.04,34.29 59.05,34.29 64.14,39.37 67.56,39.37 68.96,37.97 73.66,37.97 v73.79,37.85 | JP7.1 73.41,29.59 74.55,28.45 77.22,28.45 JP6.3
SCL5/SDO4/U2TX/PMA8/CN18/RF5  (via drill 0.23 pad 0.43)
  Top 0.127: IC3.35 28.7,30.99 v29.08,30.61 | IC2.50 58.9,24.41 v58.8,24.51
  Bottom 0.127: v29.08,30.61 32.77,30.61 33.4,29.97 38.1,29.97 42.16,25.91 47.88,25.91 49.02,27.05 53.21,27.05 53.85,27.69 54.48,27.69 54.61,27.56 56.52,27.56 58.8,25.27 v58.8,24.51
SDA1/INT4/RA15  (via drill 0.23 pad 0.43)
  Top 0.127: IC3.33 26.16,32.26 v26.29,32.38 | IC2.67 59.51,31.06 58.29,29.84 57.91,29.84 57.15,29.08 57.15,28.57 v56.64,28.07
  Bottom 0.127: R41.1 26.42,32.51 v26.29,32.38 27.3,31.37 33.02,31.37 34.04,30.35 38.48,30.35 42.55,26.29 47.5,26.29 48.64,27.43 53.09,27.43 53.72,28.07 v56.64,28.07
SDA2/RA3  (via drill 0.23 pad 0.43)
  Top 0.127: IC2.59 59.49,27.86 v59.44,27.81
  Bottom 0.127: v59.44,27.81 59.17,27.81 R19.2 | R19.2 58.93,26.42 60.2,25.15 60.2,13.21 JP4.3 | R19.2 58.42,28.07 57.53,28.07 57.4,28.19 57.4,28.57 56.9,29.08 55.75,29.08 55.5,28.83 53.59,28.83 52.96,28.19 47.62,28.19 46.48,27.05 43.31,27.05 40.89,29.46 40.89,29.59 38.23,32.26 34.16,32.26 32.51,33.91 30.48,33.91 27.18,37.21 27.18,42.93 32.38,48.13 38.99,48.13 J6.1
SDA3/SDI3/U1RX/RF2  (via drill 0.23 pad 0.43)
  Top 0.127: v57.78,24.77 57.91,24.77 58.17,25.02 60.76,25.02 IC2.52 61.55,25.06 61.85,24.77 61.85,24.26 62.74,23.37 v63.5,23.37
  Bottom 0.127: v57.78,24.77 57.78,24 56.77,22.99 51.44,22.99 50.04,24.38 41.02,24.38 38.86,26.54 22.35,26.54 21.08,25.27 21.08,22.1 20.7,21.72 19.18,21.72 18.04,20.58 R1.2 | v63.5,23.37 65.91,23.37 66.17,23.62 67.31,23.62 69.22,25.53 69.22,27.56 69.72,28.07 71.5,28.07 72.14,28.7 72.14,30.61 73.28,31.75 74.3,31.75 77.47,34.92 77.47,38.35 76.2,39.62 76.2,44.58 77.98,46.35 81.28,46.35 82.55,47.62 82.55,49.53 J9.1
SDA4/SDI2/U3RX/PMA4/CN9/RG7  (via drill 0.23 pad 0.43)
  Top 0.127: IC2.11 48.3,30.26 49.78,31.75 51.18,31.75 51.31,31.88 v51.44,31.88 | v73.15,37.08 73.15,36.83 73.91,36.07 73.91,33.27 72.26,31.62 72.26,28.32 JP6.1
  Bottom 0.127: J7.9 51.82,50.29 52.96,49.15 52.96,47.75 52.32,47.12 52.07,47.12 48.26,43.31 48.26,38.48 45.72,35.94 45.72,33.91 45.21,33.4 45.21,33.02 45.97,32.26 48.13,32.26 48.26,32.38 48.77,32.38 49.15,32 51.31,32 v51.44,31.88 51.82,31.5 56.13,31.5 57.4,32.77 57.4,33.15 58.17,33.91 59.44,33.91 61.09,35.56 61.09,35.81 62.23,36.96 62.99,36.96 65.15,39.12 67.18,39.12 68.83,37.47 72.77,37.47 v73.15,37.08 | JP7.3 80.01,28.19 80.01,26.8 79.25,26.04 74.55,26.04 JP6.1
SDA5/SDI4/U2RX/PMA9/CN17/RF4  (via drill 0.23 pad 0.43)
  Top 0.127: IC3.32 24.89,30.86 26.29,29.46 v27.81,29.46 | v57.28,25.27 57.28,24.64 57.66,24.26 58.17,24.26 58.5,23.92 IC2.49
  Bottom 0.127: v27.81,29.46 30.61,29.46 32.51,27.56 34.92,27.56 35.18,27.3 36.45,27.3 36.96,27.81 38.86,27.81 41.53,25.15 48.64,25.15 49.78,26.29 54.48,26.29 54.99,26.8 55.75,26.8 v57.28,25.27
SDO1/OC1/INT0/RD0  (via drill 0.23 pad 0.43)
  Top 0.127: IC2.72 62.02,33.06 62.87,33.91 64.01,33.91 64.64,34.54 64.64,34.92 65.28,35.56 66.42,35.56 67.06,36.2 67.06,37.85 v68.83,39.62
  Bottom 0.127: J9.7 75.06,49.66 75.06,47.24 73.91,46.1 73.91,44.7 v68.83,39.62
SS1/IC2/RD9  (via drill 0.23 pad 0.43)
  Top 0.127: IC2.69 59.96,31.86 59.82,32 v59.31,32
  Bottom 0.127: v59.31,32 59.17,32 R17.1
SS2/U6RX/U3CTS/PMA2/CN11/RG9
  Top 0.127: IC2.14 48.49,29.06 49.02,29.59 49.66,29.59 50.67,30.61 52.32,30.61 55.24,33.53 57.02,33.53 57.28,33.78 58.04,33.78 60.2,35.94 60.2,36.58 60.58,36.96 60.58,40.64 60.07,41.15 58.8,41.15 58.67,41.27 JP3.3 58.67,41.53 60.96,43.81 68.45,43.81 72.14,40.13 72.14,37.97 71.12,36.96 71.12,34.29 70.36,33.53 70.36,29.72 JP8.1 JP8.2
  Bottom 0.127: JP8.2 70.23,26.54 71.5,25.27 76.58,25.27 76.96,25.65 83.57,25.65 J10.5
SS3/U4RX/U1CTS/CN20/RD14  (via drill 0.23 pad 0.43)
  Top 0.127: IC2.47 57.7,23.58 57.53,23.75 56.77,23.75 55.88,24.64 55.88,26.04 55.12,26.8 55.12,29.84 v54.61,30.35
  Bottom 0.127: v54.61,30.35 54.23,30.73 51.31,30.73 50.8,31.24 48.39,31.24 47.88,30.73 44.83,30.73 43.94,31.62 43.94,35.81 46.74,38.61 46.74,45.72 J7.12
SS4/U5RX/U2CTS/RF12  (via drill 0.23 pad 0.43)
  Top 0.127: v13.46,32.38 IC3.23 13.5,31.71 14.22,30.99 19.18,30.99 23.11,27.05 v23.88,27.05 | IC2.40 54.9,24.55 v54.99,24.64
  Bottom 0.127: v13.46,32.38 13.46,33.01 R39.1 | v23.88,27.05 38.99,27.05 41.27,24.77 49.15,24.77 50.29,25.91 54.1,25.91 54.99,25.02 v54.99,24.64
T2CK/RC1  (via drill 0.23 pad 0.43)
  Top 0.127: IC2.6 48.26,32.26 48.39,32.38 48.64,32.38 49.15,32.89 v49.28,32.89
  Bottom 0.127: v49.28,32.89 49.66,33.27 54.1,33.27 54.74,33.91 55.63,33.91 R12.1
T3CK/RC2  (via drill 0.23 pad 0.43)
  Top 0.127: IC2.7 48.5,31.86 v48.51,31.88
  Bottom 0.127: v48.51,31.88 48.77,31.62 51.05,31.62 51.56,31.11 56.26,31.11 R13.1
T4CK/RC3  (via drill 0.23 pad 0.43)
  Top 0.127: IC2.8 48.74,31.46 49.91,32.64 v49.91,32.77
  Bottom 0.127: R14.1 54.61,32.89 50.04,32.89 v49.91,32.77
T5CK/SDI1/RC4  (via drill 0.23 pad 0.43)
  Top 0.127: IC2.9 45.9,31.06 v45.72,31.24
  Bottom 0.127: v45.72,31.24 44.83,32.13 44.83,33.66 44.7,33.78 44.7,35.18 45.34,35.81 45.34,36.2 47.75,38.61 47.75,44.2 J7.10
TCK/RA1  (via drill 0.23 pad 0.43)
  Top 0.127: IC2.38 54.1,23.62 53.98,23.75 53.72,23.75 53.47,24 53.47,30.61 55.5,32.64 v55.63,32.64 | v82.04,44.32 81.28,43.56 76.96,43.56 v72.77,39.37
  Bottom 0.127: v55.63,32.64 56.39,32.64 56.64,32.89 56.64,33.27 58.04,34.67 58.8,34.67 63.88,39.75 67.69,39.75 67.82,39.62 67.94,39.62 68.83,38.73 72.14,38.73 v72.77,39.37 | R55.1 82.05,44.33 v82.04,44.32
TDI/RA4  (via drill 0.23 pad 0.43)
  Top 0.203: IC2.60 59.62,28.26 v59.44,28.45
  Bottom 0.203: R19.1 59.32,28.57 v59.44,28.45
TDO/RA5  (via drill 0.23 pad 0.43)
  Top 0.203: IC2.61 59.98,28.66 59.69,28.96 v58.29,28.96
  Bottom 0.203: v58.29,28.96 58.29,28.95 R18.1
TMS/RA0  (via drill 0.23 pad 0.43)
  Top 0.127: IC2.17 46.53,27.86 45.97,27.3 44.2,27.3 v43.94,27.56 | v43.69,52.07 84.71,52.07 85.72,51.05 85.72,46.48 v85.09,45.85
  Bottom 0.127: v43.94,27.56 41.66,29.84 41.66,36.2 42.67,37.21 43.31,37.21 44.07,37.97 44.07,43.81 43.81,44.07 43.81,46.1 42.29,47.62 42.29,49.53 42.93,50.16 42.93,51.31 v43.69,52.07 | v85.09,45.85 R53.1
TRCLK/RA6  (via drill 0.23 pad 0.43)
  Top 0.127: IC2.91 52.9,37.01 52.7,37.21 52.7,38.48 52.2,38.99 v52.07,38.99 | v48.01,36.96 43.43,41.53 35.81,41.53 34.29,43.05 31.62,43.05 30.1,41.53 30.1,33.91 30.86,33.15 30.86,25.53 31.5,24.89 33.27,24.89 v33.78,25.4
  Bottom 0.127: v52.07,38.99 50.16,38.99 49.15,37.97 48.9,37.97 48.01,37.08 v48.01,36.96 | v33.78,25.4 R44.1
TRD0/RG13
  Top 0.127: IC2.97 50.55,36.12 50.55,35.31 50.42,35.18 49.02,35.18 48.26,35.94 47.12,35.94 46.35,36.7 45.09,36.7 40.13,31.75 40.13,24 35.31,19.18 32.13,19.18 31.62,18.67 24.38,18.67 23.62,19.43 22.35,19.43 20.83,17.91 20.83,7.75 22.61,5.97 22.61,5.13 J11.3
TRD1/RG12
  Top 0.127: IC2.96 50.9,35.15 50.55,34.8 48.77,34.8 48.13,35.43 46.99,35.43 46.35,36.07 45.09,36.07 40.89,31.88 40.89,23.62 36.07,18.8 32.38,18.8 31.62,18.03 26.42,18.03 25.91,17.53 22.6,17.53 R42.1 22.48,16.89 22.61,16.76 24.51,16.76 25.02,16.26 25.02,6.86 24.13,5.97 24.13,5.63 J11.2
TRD2/RG14
  Top 0.127: IC2.95 51.31,35.05 50.67,34.42 48.64,34.42 48.13,34.92 46.86,34.92 46.23,35.56 44.96,35.56 44.7,35.31 44.7,35.05 41.53,31.88 41.53,23.24 36.7,18.41 32.89,18.41 32,17.53 27.94,17.53 26.17,15.75 26.17,3.94 25.15,2.92 20.95,2.92 20.57,3.3 J11.5
TRD3/RA7  (via drill 0.23 pad 0.43)
  Top 0.127: IC2.92 52.5,37.03 52.32,37.21 52.32,37.97 v52.07,38.23 | v47.62,36.45 47.37,36.45 43.05,40.77 33.27,40.77 31.75,39.24 v31.75,25.65
  Bottom 0.127: v52.07,38.23 50.04,38.23 48.26,36.45 v47.62,36.45 | v31.75,25.65 31.62,25.53 25.03,25.53 R46.1
USB5V0  (via drill 0.23 pad 0.43)
  Bottom 0.127: R4.2 v10.03,27.56
  Bottom 0.254: IC1.19 13.22,26.92 C4.1 12.96,27.68 v12.95,27.69 | v12.7,29.34 12.7,28.97 C3.1 13.34,29.07 v13.34,29.34
  other vias: 6.99,26.8 6.48,27.3 8.51,27.3 7.49,27.3 8,26.8
  pour Top (no thermals): 6.22,25.91 9.02,25.91 9.02,27.43 6.22,27.43
  pour Route15 (rank 2, no thermals): 5.46,30.35 13.34,30.35 14.22,29.46 14.22,24.51 27.05,11.68 35.31,11.68 37.47,9.53 37.47,6.86 36.96,6.35 26.67,6.35 18.16,14.86 5.46,14.86
USBID/RF3  (via drill 0.23 pad 0.43)
  Top 0.127: v83.31,16.51 81.66,14.86 74.17,14.86 72.14,16.89 67.82,16.89 64.14,20.57 61.72,20.57 59.94,22.35 59.94,24.51 60.1,24.66 IC2.51
  Bottom 0.127: v83.31,16.51 83.57,16.51 83.69,16.38 84.66,16.38 J12.4
VBUS  (via drill 0.23 pad 0.43)
  Top 0.254: IC2.54 61.77,25.86 v61.85,25.78
  Bottom 0.254: v61.85,25.78 61.98,25.65 61.98,22.99 62.87,22.1 67.18,22.1 JP10.1
  other vias: 40.89,3.56 41.91,3.56 42.93,3.56 41.4,2.92 42.42,2.92 83.82,19.43 84.71,19.43 83.44,18.8 84.33,18.8 85.22,18.8
  pour Bottom (no thermals): 85.47,18.16 85.47,19.68 83.06,19.68 83.06,18.16
  pour Top (no thermals): 37.85,7.87 38.35,8.38 39.75,8.38 40.13,8 40.13,6.73 43.18,3.68 43.18,2.54 41.27,2.54 37.85,5.97
  pour Route15 (no thermals): 39.37,3.94 39.37,2.67 41.66,0.38 87.76,0.38 88.52,1.14 88.52,19.68 88.52,27.3 70.1,27.3 66.04,23.24 66.04,21.08 68.58,21.08 68.58,22.73 69.22,23.37 79.88,23.37 83.31,19.94 83.31,8.38 79.25,4.32 69.85,4.32 67.06,1.52 45.59,1.52 43.18,3.94
VCC3V3  (via drill 0.23 pad 0.43)
  Top 0.127: LD5.A v80.52,39.24 | LD6.A v78.74,39.24 | LD4.A v82.3,39.24 | LD3.A v84.07,39.24 | R42.2 v22.48,18.92
  Top 0.254: IC3.29 C23.1 v21.09,29.98 v21.08,29.97 | IC3.17 v9.65,51.56 | IC2.37 53.7,21.86 C11.1 54.48,20.58 v54.48,20.57 | v58.04,20.7 v58.03,20.71 C12.1 57.3,21.81 IC2.46 | IC2.16 46.04,28.26 C10.1 45.6,28.07 v45.21,28.07 | IC2.2 45.9,33.86 C9.1 v45.22,34.04 v45.21,34.04 | IC2.62 61.87,29.06 61.98,28.96 C13.1 63.11,28.95 v63.12,28.96 | IC2.55 62.34,26.26 C7.1 62.73,26.16 v62.99,26.16 | IC2.86 54.9,37.05 54.61,37.34 v54.61,37.47 | v21.21,3.68 21.67,4.14 J11.4
  Top 1.016: J3.2 50.8,3.05 51.94,4.19 55.37,4.19 55.63,4.45
  Bottom 0.127: R43.2 v21.09,51.3 v21.08,51.31 | R39.2 v12.45,32.52 v12.45,32.51 | R41.2 27.42,33.39 27.43,33.4 v27.43,33.53 | R7.2 v41.15,39.62 | R54.2 v80.26,16.26 | R40.2 v10.67,32.51 | R38.2 17.78,32.77 v17.78,32.51
  Bottom 0.203: D3.3 v50.93,25.4 | D4.6 68.14,9.72 v68.2,9.65 | D5.6 72.2,9.72 v72.26,9.65 | D6.6 76.14,9.72 v76.2,9.65
  Bottom 0.254: R64.2 34.29,22.35 34.04,22.61 31.88,22.61 v31.5,22.23 | C24.1 v9.64,51.55 v9.65,51.56 | D5.3 70.29,11.62 v70.36,11.68 | D4.3 v66.8,11.3 | D3.6 53.53,24.26 v53.98,24.26 | C14.1 54.35,37.2 v54.61,37.47 | D1.2 49.29,29.07 v49.28,29.08 | v17.91,49.78 17.54,49.78 C21.1 17.91,48.91 v17.91,48.9 | v3.81,34.67 3.44,34.67 C22.1 3.06,34.27 3.43,33.91 v3.81,33.91 | C25.1 21.07,3.55 v21.21,3.68
  Bottom 0.305: D6.3 73.79,11.3 v73.66,11.43
  other vias: 29.72,22.23 30.61,22.23 31.5,21.34 31.5,20.45 31.5,19.56 48.64,22.48 48.13,22.99 47.62,22.48 55.12,5.59 55.88,5.59 56.64,5.59 55.5,6.22 56.26,6.22
  pour Bottom (no thermals): 23.5,22.48 23.5,19.3 31.75,19.3 31.75,22.48
  pour Top (no thermals): 47.37,23.24 47.37,21.34 48.9,21.34 48.9,23.24
  pour Route15 (rank 3): 0,11.18 12.57,11.18 12.57,0 21.46,0 21.46,6.48 27.05,12.06 46.61,12.06 48.77,9.91 48.77,6.48 50.04,5.21 64.01,5.21 67.56,8.76 79.38,8.76 80.52,9.91 80.52,17.65 79.5,18.67 72.9,18.67 70.87,20.7 65.91,20.7 65.66,20.95 65.66,23.5 69.85,27.69 88.52,27.69 88.52,52.96 8.26,52.96 8.26,50.93 11.81,50.93 11.81,35.94 0,35.94
  pour Top (no thermals): 54.74,2.16 55.12,1.78 56.64,1.78 56.9,2.03 56.9,6.48 56.77,6.6 54.86,6.6 54.74,6.48
VCC5V0  (via drill 0.23 pad 0.43)
  other vias: 78.11,19.94 79.5,19.94 78.11,19.18 79.5,19.18
  pour Route15 (no thermals): 44.32,10.41 44.83,10.92 46.86,10.92 48.13,9.65 48.13,9.14 48.13,6.6 49.91,4.83 64.14,4.83 67.69,8.38 79.63,8.38 80.9,9.65 80.9,17.91 79.76,19.05 77.85,19.05 77.47,19.43 77.47,20.57 78.36,21.46 81.28,21.46 82.93,19.81 82.93,8.51 79.12,4.7 69.72,4.7 66.93,1.91 46.74,1.91 44.83,3.81 44.32,4.32
  pour Bottom (no thermals): 77.47,20.19 77.47,19.05 79.76,19.05 79.76,20.19
VEXT
  Top 0.889: J15.1 35.18,5.97 36.58,5.97 41.4,1.14 64.64,1.14 J3.8
  Top 1.524: J17.1 10.52,10.69 9.02,12.19 4.32,12.19 3.05,13.46 J14.1
  Bottom 1.27: J15.1 33.66,7.37 33.27,6.99 30.1,6.99 21.08,16 16.38,16 16,15.62 12.83,15.62 10.52,13.31 J17.1
  pour Top (no thermals): 9.53,9.65 9.53,5.59 10.03,5.08 10.92,5.08 11.43,5.59 11.43,9.65 10.92,10.16 10.03,10.16
  pour Bottom (no thermals): 10.03,5.08 9.53,5.59 9.53,9.65 10.03,10.16 10.92,10.16 11.43,9.65 11.43,5.59 10.92,5.08
  pour Route2 (no thermals): 9.53,9.65 10.03,10.16 10.92,10.16 11.43,9.65 11.43,5.59 10.92,5.08 10.03,5.08 9.53,5.59
  pour Route15 (no thermals): 9.53,9.65 9.53,5.59 10.03,5.08 10.92,5.08 11.43,5.59 11.43,9.65 10.92,10.16 10.03,10.16
VMON
  Bottom 0.127: 30.99,11.04 R32.2
  Bottom 0.203: R32.2 R62.2 R61.1
VREF+/CVREF+/PMA6/RA10
  Bottom 0.127: J7.15 44.07,50.8 42.67,49.4 42.67,47.75 43.94,46.48 44.44,46.48 R21.2
VREF-/CVREF-/PMA7/RA9
  Bottom 0.127: J7.16 44.2,47.74 R20.2
VRIN
  pour Bottom (rank 2, no thermals): 19.43,4.06 19.43,6.48 22.1,6.48 22.1,5.59 22.61,5.08 32.38,5.08 33.66,6.35 40.39,6.35 42.16,8.13 43.81,8.13 43.81,5.97 42.16,4.32 41.91,4.32 34.54,4.32 34.29,4.06
VROUT  (via drill 0.23 pad 0.43)
  other vias: 17.4,11.81 18.29,11.81 19.18,11.81 17.4,11.05 18.29,11.05 19.18,11.05
  pour Bottom (no thermals): 15.49,14.99 21.08,14.99 21.08,11.3 24,11.3 24,10.54 22.61,10.54 22.61,9.65 20.45,9.65 20.19,9.4 20.19,6.86 18.16,6.86 18.16,8.89 17.65,9.4 15.49,9.4
  pour Route15 (no thermals): 17.02,12.19 17.02,8.89 21.72,4.19 41.53,4.19 42.29,4.95 42.29,8.13 42.93,8.76 43.43,8.76 43.81,9.14 43.81,10.41 43.31,10.92 41.78,10.92 40.51,9.65 40.51,7.24 39.24,5.97 26.42,5.97 17.78,14.61 17.02,14.61
VU
  Bottom 0.254: J15.2 33.27,9.91 32.64,9.27 32.38,9.27 R61.2
  pour Bottom (no thermals): 32.77,10.29 32.77,9.4 33.4,8.76 39.24,8.76 39.62,8.38 43.94,8.38 44.45,7.87 44.45,6.73 44.83,6.35 46.1,6.35 46.48,6.73 46.48,9.02 43.94,11.56 34.04,11.56
  pour Bottom (rank 2, no thermals): 37.08,16.89 37.08,14.99 34.92,14.99 34.8,14.86 34.8,11.81 35.05,11.56 35.05,10.92 33.4,10.92 33.4,14.99 33.02,14.99 33.02,16.89

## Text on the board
tPlace: 1 | SCL | SDA | A | G | 9 | 8 | 7 | 6 | 5 | 4 | 3 | 2 | 1 | 0 | 13 | 12 | 11 | 10 | TX | RX | 31 | 30 | 41 | 40 | 39 | 38 | 37 | 36 | 35 | 34 | 33 | 32 | 29 | 28 | 27 | 26 | 1 | PWM | 10 | SS | GND | RESET | (AN13) | SPI | MASTER | SLAVE | 1 | SPI | SELECT | ICSP | 1 | 1 | USB | UART | AB | A | 1 | GND | VU SELECT | + | - | AN | I2C | 15V MAX! | EXT | UART | USB | LDO | OUT | 5V0 | GND | 1 | A6 | A7 | A8 | A10 | A11 | A0 | A1 | A2 | A3 | A9 | A4 | A5 | 1 | 1 | EN | ANALOG | IN | VU | EXT | IOREF | RST | 3V3 | 5V0 | GND | GND | VIN | LDO | + | _
bPlace: PB200-273 | REV B
Measures: Slot Drills | 0.026 x 0.125"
